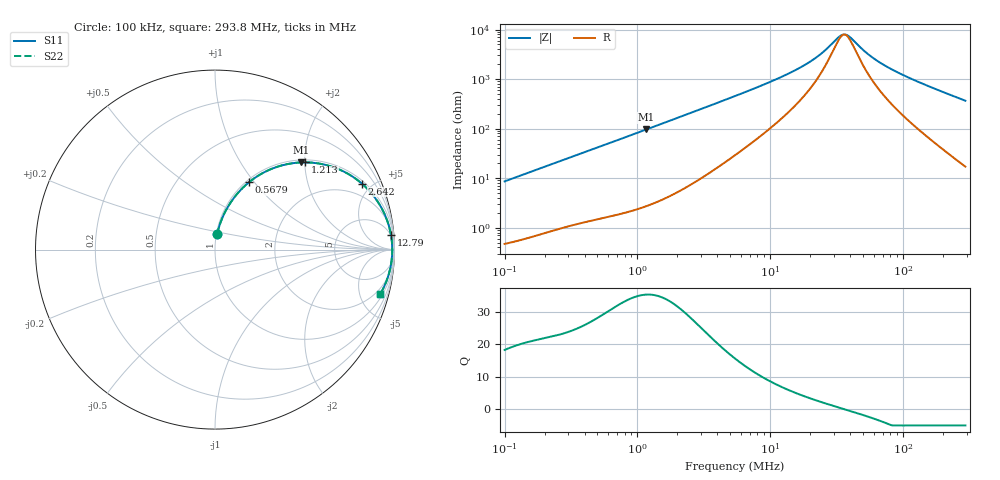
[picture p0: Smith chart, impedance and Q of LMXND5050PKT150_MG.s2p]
! LMXND5050PKT150_MG  S-PARAMETER MODEL  ( General Type )
! Model Generated by TAIYO YUDEN Corporation (http://www.ty-top.com)
! Version 1.0
! TAIYO YUDEN Control No. 191023NI43SB-FBB
! Copyright(c) 2019 TAIYO YUDEN CO.,LTD. All Rights Reserved.
! Product Description (link to TY-COMPAS)
! https://ds.yuden.co.jp/TYCOMPAS/or/detail?pn=LMXND5050PKT150MMG&u=M
! Products Name : Inductors
! Characteristics :
!  Inductance : 15 uH , SRF(min) : 20 MHz , DC Resistance(max) : 0.384 Ohm
!  Rated Current : Saturation :1100 mA , Temp Rise : 650 mA
!  Case Size : 4.9 x 4.9 / 0.193 x 0.193 [mm/inch] , Thickness : 1.4 / 0.055 [mm/inch]
!  (Conditions: Temperature = 25 degC , DC Bias Current/Voltage = 0A / 0V)
! External Node Assignments :
!  1  o---GGG---o  2
! GND o---------o GND
! Frequency Range : 0.1MHz  -  293.796821MHz  [ 402 STEP ]
# MHz S RI R 50
! Freq[MHz].  S11 Real  S11 Imag  S21 Real  S21 Imag  S12 Real  S12 Imag  S22 Real  S22 Imag
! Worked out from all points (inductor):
!   401 points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, 100 kHz to 293.8 MHz, reference 50 ohm
!   read as one part in series: L = 13.7 uH near 104.1 kHz
!   highest Q = 35.3 at 1.165 MHz (marker M1), where L = 13.1 uH
!   self-resonance near 36.04 MHz
!   S11 on the Smith chart (normalised r, x): 100 kHz: 1.01, +0.17; 567.9 kHz: 1.03, +0.94; 1.213 MHz: 1.06, +2.00; 2.642 MHz: 1.16, +4.37; 12.79 MHz: 5, +23; 293.8 MHz: 1.34, -7.32
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0.1  0.012 0.0848  0.988 -0.0848  0.988 -0.0848  0.012 0.0848
0.197144  0.0345 0.1609  0.9655 -0.1609  0.9655 -0.1609  0.0345 0.1609
0.380976  0.1017 0.2832  0.8983 -0.2832  0.8983 -0.2832  0.1017 0.2832
0.567937  0.1905 0.3761  0.8095 -0.3761  0.8095 -0.3761  0.1905 0.3761
0.846647  0.334 0.457  0.666 -0.457  0.666 -0.457  0.334 0.457
1.165264  0.4815 0.4857  0.5185 -0.4857  0.5185 -0.4857  0.4815 0.4857
1.212732  0.5008 0.486  0.4992 -0.486  0.4992 -0.486  0.5008 0.486
1.451429  0.587 0.4782  0.413 -0.4782  0.413 -0.4782  0.587 0.4782
2.641796  0.818 0.368  0.182 -0.368  0.182 -0.368  0.818 0.368
3.709294  0.8938 0.2856  0.1062 -0.2856  0.1062 -0.2856  0.8938 0.2856
5.420303  0.942 0.2039  0.058 -0.2039  0.058 -0.2039  0.942 0.2039
12.78906  0.9806 0.0808  0.0194 -0.0808  0.0194 -0.0808  0.9806 0.0808
20.65007  0.9859 0.0387  0.0141 -0.0387  0.0141 -0.0387  0.9859 0.0387
25.21289  0.9869 0.0241  0.0131 -0.0241  0.0131 -0.0241  0.9869 0.0241
32.68392  0.9875 0.00647  0.0125 -0.00647  0.0125 -0.00647  0.9875 0.00647
36.11476  0.9876 -0.000146  0.0124 0.000146  0.0124 0.000146  0.9876 -0.000146
39.90573  0.9876 -0.00677  0.0124 0.00677  0.0124 0.00677  0.9876 -0.00677
49.70575  0.9871 -0.0217  0.0129 0.0217  0.0129 0.0217  0.9871 -0.0217
58.31329  0.9865 -0.0331  0.0135 0.0331  0.0135 0.0331  0.9865 -0.0331
78.67184  0.9843 -0.057  0.0157 0.057  0.0157 0.057  0.9843 -0.057
137.5887  0.9738 -0.1161  0.0262 0.1161  0.0262 0.1161  0.9738 -0.1161
293.7968  0.9207 -0.2479  0.0793 0.2479  0.0793 0.2479  0.9207 -0.2479
